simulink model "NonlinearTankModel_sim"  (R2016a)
settings: Solver=VariableStepAuto  StartTime=0.0  StopTime=Endtime  RelTol=1e-3
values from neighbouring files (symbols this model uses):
  C = D^2/4*pi    (= 0.196349540849)    [NonlinearTankModel.m]    (also in TankModel.m; RLCModel.m = 0.0001; TempModel.m = 4187; TankModel_with_Sensor.m)
  g = 9.8    [NonlinearTankModel.m]    (also in MSDModel.m)
  q1 = 1e-3:1e-3:5e-3    [NonlinearTankModel.m]    (also in TankModel.m = 0.001; TempModel.m = 300)
  Z = 1e-3    (= 0.001)    [NonlinearTankModel.m]

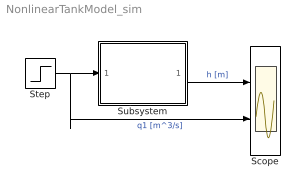
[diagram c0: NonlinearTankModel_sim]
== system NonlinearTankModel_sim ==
  Scope : Scope  NumInputPorts=2
  Step : Step  After=q1  SampleTime=0
  Subsystem : Subsystem
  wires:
  Step/1 -> Scope/2, Subsystem/1(q [m^3/s])  "q1 [m^3/s]"
  Subsystem/1(h [m]) -> Scope/1  "h [m]"

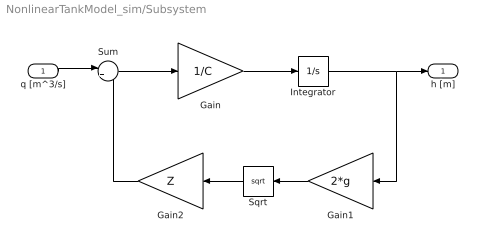
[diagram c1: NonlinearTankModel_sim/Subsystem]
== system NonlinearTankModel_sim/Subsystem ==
  q [m^3/s] : Inport
  Gain : Gain  Gain=1/C
  Gain1 : Gain  Gain=2*g
  Gain2 : Gain  Gain=Z
  Integrator : Integrator
  Sqrt : Sqrt
  Sum : Sum  Inputs=|+-
  h [m] : Outport
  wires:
  Sqrt/1 -> Gain2/1
  Gain/1 -> Integrator/1
  Gain1/1 -> Sqrt/1
  Sum/1 -> Gain/1
  Integrator/1 -> h [m]/1, Gain1/1
  Gain2/1 -> Sum/2
  q [m^3/s]/1 -> Sum/1
